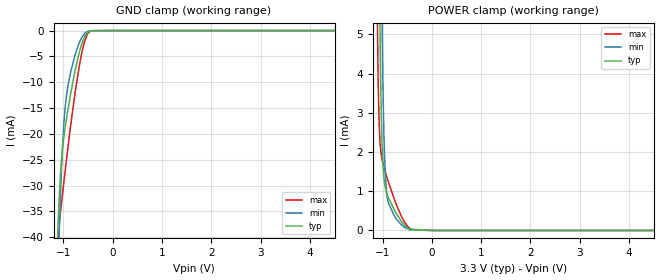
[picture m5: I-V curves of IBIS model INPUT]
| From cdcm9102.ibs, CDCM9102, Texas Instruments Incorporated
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|   INPUT
[Model]   INPUT
Model_type   Input
| Signals   CE,OS1,OS0,RSTN,OD0,OD1,OD2,PR0,PR1
Vinl = 1.32V
Vinh = 1.98V
| variable   typ   min   max
C_comp   0.754pF   0.736pF   0.781pF
[Temperature Range]   40.0   100.0   -40.0
[Voltage range]   3.3V   3.0V   3.6V
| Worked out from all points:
|   GND clamp passes 1 mA (typ) near -0.56 V on its own axis
|   POWER clamp passes 1 mA (typ) near -0.93 V on its own axis
[GND Clamp]
|   Voltage   I(typ)   I(min)   I(max)
-3.3V     -1.078A    -1.09A     -1.066A
-1.119V   -40.67mA   -50.59mA   -41.17mA
-1.089V   -33.4mA    -40.8mA    -38.05mA
-1.075V   -30.47mA   -36.36mA   -36.65mA
-1.048V   -26.2mA    -29.03mA   -34.21mA
-995.6mV  -20.97mA   -18.75mA   -29.75mA
-926.1mV  -16.37mA   -11.8mA    -24.07mA
-832.1mV  -11.18mA   -7.252mA   -16.9mA
-701mV    -5.142mA   -2.948mA   -8.24mA
-609.2mV  -2.076mA   -1.048mA   -3.57mA
-515.3mV  -441.4uA   -214.5uA   -756.5uA
6.598V    0A         0A         0A
[POWER Clamp]
|   Voltage   I(typ)   I(min)   I(max)
-3.3V     1.053A     1.062A     1.045A
-1.104V   14.54mA    25.31mA    5.321mA
-1.075V   8.309mA    17.09mA    2.962mA
-1.052V   5.139mA    11.97mA    2.272mA
-1.035V   3.531mA    8.762mA    2.014mA
-1.015V   2.39mA     5.923mA    1.841mA
-1.005V   2.016mA    4.81mA     1.777mA
-993mV    1.686mA    3.713mA    1.709mA
-960.8mV  1.217mA    1.929mA    1.559mA
-913.8mV  941uA      930uA      1.362mA
-473.3mV  49.73uA    28.36uA    76.32uA
6.598V    0A         0A         0A
